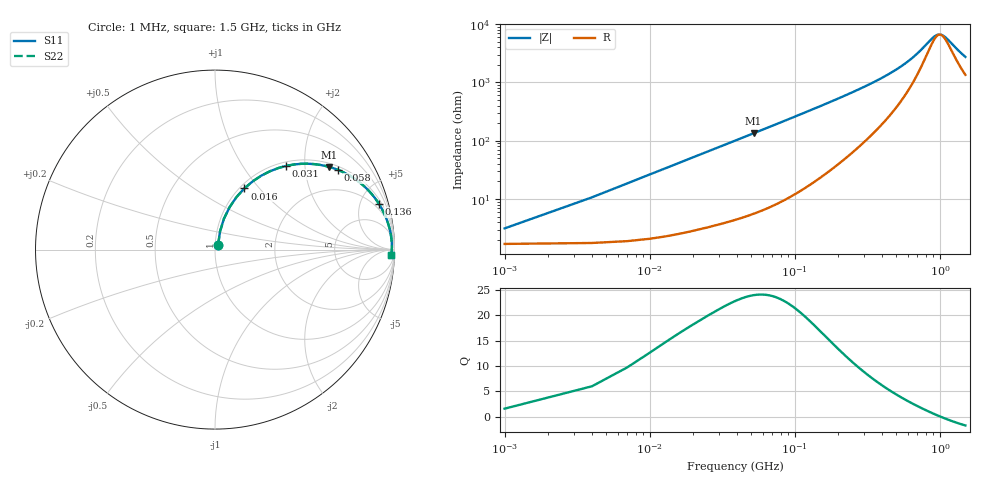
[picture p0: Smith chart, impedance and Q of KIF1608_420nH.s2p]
# MHz S RI R 50
!Freq ReS11 ImS11 ReS21 ImS21 ReS12 ImS12 ReS22 ImS22
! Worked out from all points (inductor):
!   501 points, 1 MHz to 1.5 GHz, reference 50 ohm
!   read as one part in series: L = 418 nH near 7 MHz
!   highest Q = 24 at 52 MHz (marker M1), where L = 410 nH
!   self-resonance near 1.004 GHz
!   S11 on the Smith chart (normalised r, x): 1 MHz: 1.03, +0.05; 16 MHz: 1.05, +0.84; 31 MHz: 1.07, +1.60; 58 MHz: 1.12, +2.99; 136 MHz: 1.39, +7.07; 1.5 GHz: 28, -48
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1  0.0174 0.0255  0.9826 -0.0255  0.9826 -0.0255  0.0174 0.0255
4  0.0278 0.1008  0.9722 -0.1008  0.9722 -0.1008  0.0278 0.1008
10  0.0812 0.2364  0.9188 -0.2364  0.9188 -0.2364  0.0812 0.2364
13  0.12 0.293  0.88 -0.293  0.88 -0.293  0.12 0.293
16  0.1638 0.341  0.8362 -0.341  0.8362 -0.341  0.1638 0.341
22  0.2582 0.412  0.7418 -0.412  0.7418 -0.412  0.2582 0.412
31  0.3968 0.4665  0.6032 -0.4665  0.6032 -0.4665  0.3968 0.4665
40  0.5156 0.4785  0.4844 -0.4785  0.4844 -0.4785  0.5156 0.4785
52  0.637 0.4605  0.363 -0.4605  0.363 -0.4605  0.637 0.4605
58  0.6838 0.4447  0.3162 -0.4447  0.3162 -0.4447  0.6838 0.4447
88  0.827 0.3567  0.173 -0.3567  0.173 -0.3567  0.827 0.3567
136  0.9142 0.2537  0.0858 -0.2537  0.0858 -0.2537  0.9142 0.2537
190  0.9497 0.1856  0.0503 -0.1856  0.0503 -0.1856  0.9497 0.1856
253  0.9669 0.138  0.0331 -0.138  0.0331 -0.138  0.9669 0.138
355  0.978 0.0929  0.022 -0.0929  0.022 -0.0929  0.978 0.0929
502  0.9835 0.0566  0.0165 -0.0566  0.0165 -0.0566  0.9835 0.0566
751  0.9856 0.0222  0.0144 -0.0222  0.0144 -0.0222  0.9856 0.0222
904  0.9855 0.00794  0.0145 -0.00794  0.0145 -0.00794  0.9855 0.00794
1003  0.9852 9.68e-05  0.0148 -9.68e-05  0.0148 -9.68e-05  0.9852 9.68e-05
1084  0.9847 -0.00574  0.0153 0.00574  0.0153 0.00574  0.9847 -0.00574
1252  0.9836 -0.0166  0.0164 0.0166  0.0164 0.0166  0.9836 -0.0166
1500  0.9814 -0.0306  0.0186 0.0306  0.0186 0.0306  0.9814 -0.0306
